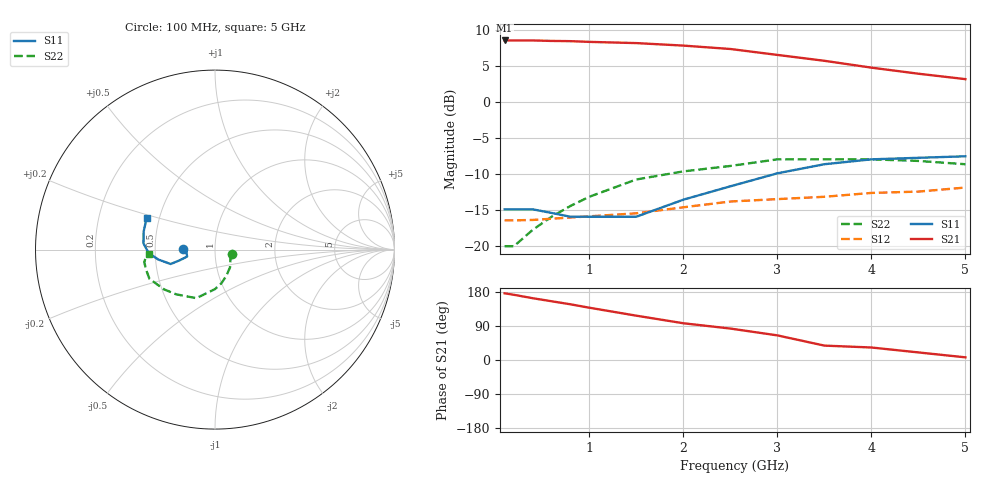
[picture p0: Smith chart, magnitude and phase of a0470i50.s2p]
!  MSA-0470 S AND NOISE PARAMETERS
!  Id=50mA  LAST UPDATED 07-22-92
# ghz s ma r 50
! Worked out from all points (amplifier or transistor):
!   14 points, 100 MHz to 5 GHz, reference 50 ohm
!   highest |S21| = 8.5 dB at 100 MHz (marker M1)
!   |S21| within 3 dB of that: start of sweep to 3.595 GHz
!   unconditionally stable (mu >= 1): start of sweep to 2.696 GHz; 4.841 GHz to end of sweep
!   at 400 MHz: K = 1.36, MAG = 8.9 dB, |S12| = -16.4 dB
!   at 2 GHz: K = 1.11, MAG = 9.2 dB, |S12| = -14.6 dB
!   at 5 GHz: K = 1.01, MAG = 7.0 dB, |S12| = -11.9 dB
!   lowest NFmin = 6.10 dB at 100 MHz
0.1  0.18 179.0  2.67 176.0  0.151 1.0  0.1 -14.0
0.2  0.18 179.0  2.67 172.0  0.151 2.0  0.1 -30.0
0.4  0.18 179.0  2.67 163.0  0.152 3.0  0.13 -50.0
0.6  0.17 -179.0  2.65 155.0  0.155 5.0  0.16 -67.0
0.8  0.16 -176.0  2.64 147.0  0.158 6.0  0.19 -79.0
1  0.16 -174.0  2.61 138.0  0.161 6.0  0.22 -90.0
1.5  0.16 -166.0  2.56 117.0  0.169 9.0  0.29 -111.0
2  0.21 -163.0  2.46 97.0  0.186 9.0  0.33 -131.0
2.5  0.26 -162.0  2.33 83.0  0.204 12.0  0.36 -142.0
3  0.32 -170.0  2.12 65.0  0.212 10.0  0.4 -156.0
3.5  0.37 -177.0  1.93 38.0  0.22 7.0  0.4 -164.0
4  0.4 175.0  1.73 33.0  0.234 3.0  0.4 -170.0
4.5  0.41 166.0  1.57 20.0  0.239 -1.0  0.39 -173.0
5  0.42 155.0  1.44 7.0  0.255 -6.0  0.37 -176.0
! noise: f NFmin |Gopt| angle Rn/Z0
0.1  6.1  0.13  179  0.64
0.5  6.1  0.13  178  0.64
1  6.4  0.15  179  0.64
2  7.2  0.19  -172  0.62
